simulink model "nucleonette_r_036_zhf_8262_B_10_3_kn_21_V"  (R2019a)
settings: Solver=VariableStepAuto  StartTime=0.0  StopTime=727544.216  FixedStep=0.2  RelTol=1e-6
libraries: simulink x6
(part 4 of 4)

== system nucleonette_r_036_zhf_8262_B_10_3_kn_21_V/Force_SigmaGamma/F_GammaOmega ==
  In1 : Inport
  Add31 : Sum  Inputs=+++
  Add40 : Sum
  Add51 : Sum
  C_10 : Constant  Value=10
  C_100 : Constant  Value=-100
  C_10_11 : Constant  Value=1E-21
  Clock1 : Clock
  Constant : Constant  Value=3
  Constant1 : Constant  Value=2
  Constant15 : Constant  Value=1.0E-3
  Constant24 : Constant  Value=3
  Math Function{1,4,27,30} (4 alike) : Math  Operator=square
  Math Function32 : Math  Operator=pow
  Math Function37 : Math  Operator=pow
  Math Function45 : Math  Operator=pow
  NGamOmex/DGamOmex_3 : Scope
  Omega_w1 : Constant  Value=0.00003453723537
  Product1 : Product  Inputs=*/
  Product{3..4,6..7,12,45,57..58,60} (9 alike) : Product
  Product2 : Product  Inputs=*/
  Product26 : Product  Inputs=*/
  Product31 : Product  Inputs=/**
  Product33 : Product  Inputs=/**
  Product44 : Product  Inputs=**
  Sqrt13 : Sqrt
  Sqrt4 : Sqrt
  Subtract3 : Sum  Inputs=+--
  Subtract4 : Sum
  Trigonometric Function9 : Trigonometry
  ex : Constant  Value=1.602176565
  keGamOmex : Constant  Value=7.39283526
  mSigGamx : Constant  Value=366.300038182
  rx1 : Constant  Value=0.36373
  Out1 : Outport
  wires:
  Math Function1/1 -> Add31/2  "XGO"
  Subtract3/1 -> Product60/2  "Zx_GamOme"
  Product1/1 -> Product3/1, Product7/1  "3/2"
  Omega_w1/1 -> Product57/2
  rx1/1 -> Subtract4/2, Product6/2, Product4/2, Product33/1  "rx"
  Product33/1 -> Math Function37/2
  Math Function32/1 -> Add51/2
  Math Function45/1 -> Add51/1
  Product60/1 -> Product26/1
  C_10/1 -> Math Function37/1
  Constant24/1 -> Math Function45/2, Math Function32/2
  Product57/1 -> Trigonometric Function9/1  "angle_wt"
  Trigonometric Function9/1 -> Product4/1  "sin(wt)"
  Product31/1 -> Product45/2
  Product58/1 -> Math Function27/1  "r*sin(wt)*sqrt(3)/2"
  Product6/1 -> Subtract3/2  "r*sqrt(3)/2"
  Math Function4/1 -> Product31/2
  Product26/1 -> Out1/1, NGamOmex/DGamOmex_3/1  "F_GamOme"
  Clock1/1 -> Product57/1
  Add51/1 -> Product26/2  "DGamOme_B"
  Product45/1 -> Product60/1
  Product4/1 -> Product58/2, Product7/2, Product12/1  "r*sin(wt)"
  Sqrt4/1 -> Product33/2, Math Function32/1  "DGamOme"
  Constant15/1 -> Math Function45/1
  ex/1 -> Math Function4/1
  Constant1/1 -> Product1/2, Product2/2
  Subtract4/1 -> Math Function30/1  "YGamOme"
  Product3/1 -> Subtract3/3  "3z6/2"
  mSigGamx/1 -> Product31/1  "mx"
  Product2/1 -> Product58/1, Product6/1, Product12/2  "sqrt(3)/2"
  Add40/1 -> Product45/1  "kn_DGamOme"
  Constant/1 -> Product1/1, Sqrt13/1
  Math Function37/1 -> Add40/1  "10_exp(-100Dgo/r)"
  C_100/1 -> Product33/3
  Sqrt13/1 -> Product44/2, Product2/1  "sqrt(3)"
  Product12/1 -> Subtract3/1  "r*sin(wt)*sqrt(3)/2"
  C_10_11/1 -> Add40/2
  In1/1 -> Product3/2, Product44/1  "z6"
  Math Function30/1 -> Add31/3
  keGamOmex/1 -> Product31/3
  Math Function27/1 -> Add31/1  "ZGO"
  Add31/1 -> Sqrt4/1
  Product7/1 -> Math Function1/1  "r*sin(wt)3/2"
  Product44/1 -> Subtract4/1  "z6*sqrt(3)"

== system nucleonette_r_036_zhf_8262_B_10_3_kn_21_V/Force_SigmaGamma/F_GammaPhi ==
  In1 : Inport
  Add31 : Sum  Inputs=+++
  Add40 : Sum
  Add51 : Sum
  C_10 : Constant  Value=10
  C_100 : Constant  Value=-100
  C_10_11 : Constant  Value=1E-21
  Clock1 : Clock
  Constant : Constant  Value=3
  Constant1 : Constant  Value=2
  Constant15 : Constant  Value=1.0E-3
  Constant24 : Constant  Value=3
  Math Function{1,4,27,30} (4 alike) : Math  Operator=square
  Math Function32 : Math  Operator=pow
  Math Function37 : Math  Operator=pow
  Math Function45 : Math  Operator=pow
  NGamPhix/DGamPhix_3 : Scope
  Omega_w1 : Constant  Value=0.00003453723537
  Product1 : Product  Inputs=*/
  Product{3..6,12,45,57..58,60} (9 alike) : Product
  Product2 : Product  Inputs=*/
  Product26 : Product  Inputs=*/
  Product31 : Product  Inputs=/**
  Product33 : Product  Inputs=/**
  Product44 : Product  Inputs=**
  Sqrt13 : Sqrt
  Sqrt4 : Sqrt
  Subtract3 : Sum  Inputs=+++
  Subtract4 : Sum  Inputs=+++
  Trigonometric Function10 : Trigonometry  Operator=cos
  Trigonometric Function9 : Trigonometry
  ex : Constant  Value=1.602176565
  keGamPhix : Constant  Value=7.39283526
  mSigGamx : Constant  Value=366.300038182
  rx1 : Constant  Value=0.36373
  Out1 : Outport
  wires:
  Product12/1 -> Subtract3/1  "r*sin(wt)*sqrt(3)/2"
  C_100/1 -> Product33/3
  Constant/1 -> Product1/1, Sqrt13/1
  mSigGamx/1 -> Product31/1  "mx"
  Product3/1 -> Subtract3/3  "3z6/2"
  Subtract4/1 -> Math Function30/1  "YGamPhi"
  Constant1/1 -> Product1/2, Product2/2
  ex/1 -> Math Function4/1
  Constant15/1 -> Math Function45/1
  Sqrt4/1 -> Product33/2, Math Function32/1  "DGamPhi"
  Product4/1 -> Subtract4/1, Product12/1  "r*sin(wt)"
  Product2/1 -> Product6/1, Product12/2  "sqrt(3)/2"
  Product45/1 -> Product60/1
  Add51/1 -> Product26/2  "DGamPhi_B"
  Clock1/1 -> Product57/1
  Product26/1 -> Out1/1, NGamPhix/DGamPhix_3/1  "F_GamPhi"
  Math Function4/1 -> Product31/2
  Product6/1 -> Subtract3/2  "r*sqrt(3)/2"
  Product58/1 -> Math Function27/1  "r*cos(wt)*sqrt(3)"
  Omega_w1/1 -> Product57/2
  Product1/1 -> Product3/1  "3/2"
  Subtract3/1 -> Product60/2  "Zx_GamPhi"
  Math Function1/1 -> Add31/2  "XGP"
  Product33/1 -> Math Function37/2
  Math Function32/1 -> Add51/2
  rx1/1 -> Subtract4/3, Product5/2, Product6/2, Product4/2, Product33/1  "rx"
  Math Function37/1 -> Add40/1  "10_exp(-100Dgp/r)"
  C_10_11/1 -> Add40/2
  Math Function45/1 -> Add51/1
  Add40/1 -> Product45/1  "kn_DGamPhi"
  C_10/1 -> Math Function37/1
  Sqrt13/1 -> Product58/1, Product44/2, Product2/1  "sqrt(3)"
  Product60/1 -> Product26/1
  Math Function27/1 -> Add31/1  "ZGP"
  Trigonometric Function10/1 -> Product5/1  "cos(wt)"
  Math Function30/1 -> Add31/3
  Constant24/1 -> Math Function32/2, Math Function45/2
  In1/1 -> Product3/2, Product44/1  "z6"
  Trigonometric Function9/1 -> Product4/1  "sin(wt)"
  Product31/1 -> Product45/2
  Add31/1 -> Sqrt4/1
  Product57/1 -> Trigonometric Function10/1, Trigonometric Function9/1  "angle_wt"
  keGamPhix/1 -> Product31/3
  Product5/1 -> Product58/2, Math Function1/1  "r*cos(wt)"
  Product44/1 -> Subtract4/2  "z6*sqrt(3)"

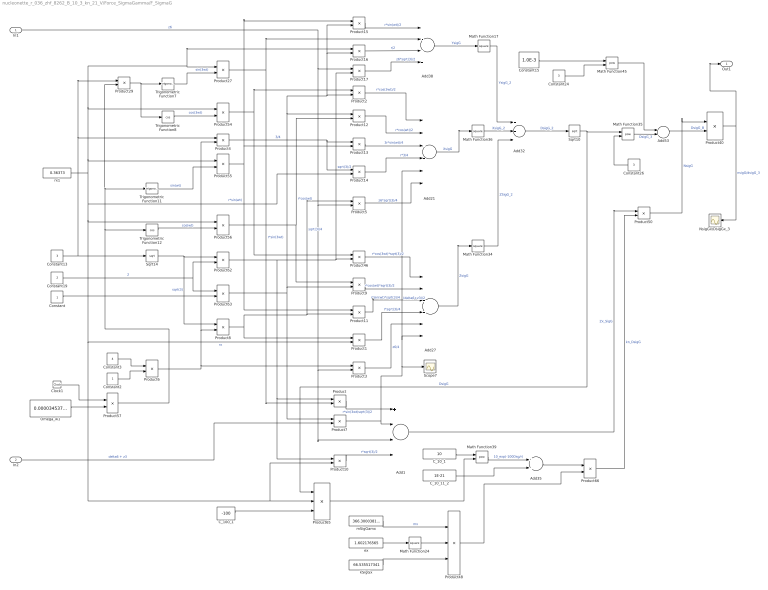
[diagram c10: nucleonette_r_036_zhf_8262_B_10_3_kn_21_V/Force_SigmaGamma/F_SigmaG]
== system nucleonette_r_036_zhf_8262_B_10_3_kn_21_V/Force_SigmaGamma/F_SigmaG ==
  In1 : Inport
  In2 : Inport  Port=2
  Add1 : Sum  Inputs=+---
  Add21 : Sum  Inputs=-+----
  Add27 : Sum  Inputs=-+++++
  Add32 : Sum  Inputs=+++
  Add35 : Sum
  Add38 : Sum  Inputs=--++
  Add53 : Sum
  C_100_1 : Constant  Value=-100
  C_10_1 : Constant  Value=10
  C_10_11_2 : Constant  Value=1E-21
  Clock1 : Clock
  Constant : Constant
  Constant13 : Constant  Value=3
  Constant15 : Constant  Value=1.0E-3
  Constant19 : Constant  Value=2
  Constant2 : Constant
  Constant24 : Constant  Value=3
  Constant26 : Constant  Value=3
  Constant3 : Constant  Value=4
  Math Function{17,24,34,36} (4 alike) : Math  Operator=square
  Math Function35 : Math  Operator=pow
  Math Function39 : Math  Operator=pow
  Math Function45 : Math  Operator=pow
  NsigGx/DsigGx_3 : Scope
  Omega_w1 : Constant  Value=0.00003453723537
  Product{,1..5,7..17,29,46,50,57} (21 alike) : Product
  Product{27,54..56,66} (5 alike) : Product  Inputs=**
  Product40 : Product  Inputs=*/
  Product48 : Product  Inputs=/**
  Product6 : Product  Inputs=/*
  Product62 : Product  Inputs=*/
  Product63 : Product  Inputs=/*
  Product65 : Product  Inputs=*/*
  Scope7 : Scope
  Sqrt10 : Sqrt
  Sqrt14 : Sqrt
  Trigonometric Function11 : Trigonometry
  Trigonometric Function12 : Trigonometry  Operator=cos
  Trigonometric Function7 : Trigonometry
  Trigonometric Function8 : Trigonometry  Operator=cos
  ex : Constant  Value=1.602176565
  kSigGx : Constant  Value=66.535517341
  mSigGamx : Constant  Value=366.300038182
  rx1 : Constant  Value=0.36373
  Out1 : Outport
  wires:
  Add32/1 -> Sqrt10/1  "DsigG_2"
  Add1/1 -> Product50/1  "Zx_SigG"
  Product46/1 -> Add27/1  "r*cos(3wt)*sqrt(3)/2"
  Product62/1 -> Product10/1, Product/1, Product17/2, Product46/2  "sqrt(3)/2"
  Product/1 -> Add1/1  "r*sin(3wt)sqrt(3)/2"
  Product9/1 -> Add27/2  "r*cos(wt)*sqrt(3)/2"
  Math Function45/1 -> Add53/1
  Product29/1 -> Trigonometric Function8/1, Trigonometric Function7/1
  Add53/1 -> Product40/2  "DsigG_B"
  Add27/1 -> Math Function34/1  "ZsigG"
  Product8/1 -> Product11/2, Product5/1, Product1/1  "sqrt(3)/4"
  Constant3/1 -> Product6/1
  Product1/1 -> Add27/4  "r*sqrt(3)/4"
  Add38/1 -> Math Function17/1  "YsigG"
  Product11/1 -> Add27/3  "r*sin(wt)*sqrt(3)/4"
  Product56/1 -> Product12/2, Product9/1  "r*cos(wt)"
  Math Function34/1 -> Add32/3  "ZSigG_2"
  Product55/1 -> Product15/1, Product13/2, Product11/1  "r*sin(wt)"
  Product48/1 -> Product66/2
  Math Function36/1 -> Add32/2  "XsigG_2"
  Constant26/1 -> Math Function35/2
  Product63/1 -> Product12/1, Product2/2, Product15/2, Product16/2, Product9/2, Product7/1
  Product2/1 -> Add21/1  "r*cos(3wt)/2"
  Add35/1 -> Product66/1
  Product13/1 -> Add21/3  "3r*sin(wt)/4"
  Omega_w1/1 -> Product57/2
  Math Function17/1 -> Add32/1  "YsigG_2"
  Product5/1 -> Add21/6  "z6*sqrt(3)/4"
  Product54/1 -> Product2/1, Product46/1
  Product66/1 -> Product50/2  "kn_DsigG"
  Math Function39/1 -> Add35/1  "10_exp(-100Dsg/r)"
  Product12/1 -> Add21/2  "r*cos(wt)/2"
  Product14/1 -> Add21/4  "r*3/4"
  Constant13/1 -> Product4/1, Product29/1, Sqrt14/1
  Trigonometric Function8/1 -> Product54/2  "cos(3wt)"
  In2/1 -> Product7/2  "delta6 + z3"
  Trigonometric Function7/1 -> Product27/2  "sin(3wt)"
  Product7/1 -> Add1/2, Scope7/1, Add21/5, Add27/6  "(delta6+z3)/2"
  Trigonometric Function12/1 -> Product56/2  "cos(wt)"
  Math Function35/1 -> Add53/2  "DsigG_3"
  Product16/1 -> Add38/3  "r/2"
  Product6/1 -> Product4/2, Product8/2, Product3/1
  Product15/1 -> Add38/1  "r*sin(wt)/2"
  Constant19/1 -> Product63/1, Product62/2  "2"
  Product17/1 -> Add38/4  "z6*sqrt(3)/2"
  In1/1 -> Add1/3, Product3/2, Product5/2, Product17/1  "z6"
  Product3/1 -> Add27/5  "z6/4"
  Sqrt10/1 -> Product65/1, Math Function35/1  "DsigG"
  mSigGamx/1 -> Product48/1  "mx"
  Product40/1 -> NsigGx/DsigGx_3/1, Out1/1  "nsigG/dsigG_3"
  Math Function24/1 -> Product48/2
  Trigonometric Function11/1 -> Product55/2  "sin(wt)"
  Product65/1 -> Math Function39/2
  Constant15/1 -> Math Function45/1
  Constant24/1 -> Math Function45/2
  kSigGx/1 -> Product48/3
  Product4/1 -> Product13/1, Product14/1  "3/4"
  rx1/1 -> Product16/1, Product27/1, Product54/1, Product55/1, Product14/2, Product1/2, Product10/2, Product65/2, Product56/1  "rx"
  ex/1 -> Math Function24/1
  Product27/1 -> Add38/2, Product/2  "r*sin(3wt)"
  Product50/1 -> Product40/1  "NsigG"
  C_10_1/1 -> Math Function39/1
  Constant/1 -> Product63/2
  Product57/1 -> Trigonometric Function12/1, Product29/2, Trigonometric Function11/1
  Clock1/1 -> Product57/1
  C_10_11_2/1 -> Add35/2
  C_100_1/1 -> Product65/3
  Add21/1 -> Math Function36/1  "XsigG"
  Sqrt14/1 -> Product62/1, Product8/1  "sqrt(3)"
  Constant2/1 -> Product6/2
  Product10/1 -> Add1/4  "r*sqrt(3)/2"

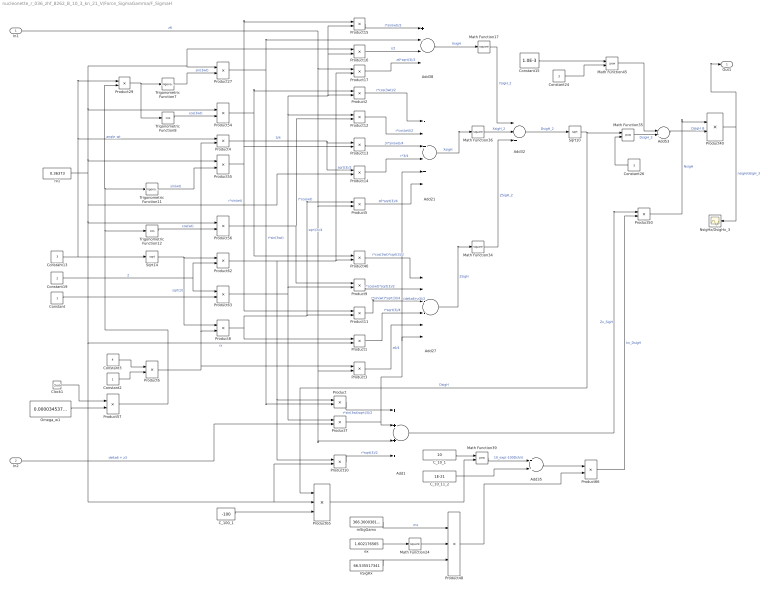
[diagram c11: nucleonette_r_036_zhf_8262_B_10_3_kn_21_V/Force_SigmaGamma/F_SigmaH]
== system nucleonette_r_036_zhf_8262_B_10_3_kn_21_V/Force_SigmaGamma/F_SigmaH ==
  In1 : Inport
  In2 : Inport  Port=2
  Add1 : Sum  Inputs=++++
  Add21 : Sum  Inputs=--++++
  Add27 : Sum  Inputs=------
  Add32 : Sum  Inputs=+++
  Add35 : Sum
  Add38 : Sum  Inputs=+---
  Add53 : Sum
  C_100_1 : Constant  Value=-100
  C_10_1 : Constant  Value=10
  C_10_11_2 : Constant  Value=1E-21
  Clock1 : Clock
  Constant : Constant
  Constant13 : Constant  Value=3
  Constant15 : Constant  Value=1.0E-3
  Constant19 : Constant  Value=2
  Constant2 : Constant
  Constant24 : Constant  Value=3
  Constant26 : Constant  Value=3
  Constant3 : Constant  Value=4
  Math Function{17,24,34,36} (4 alike) : Math  Operator=square
  Math Function35 : Math  Operator=pow
  Math Function39 : Math  Operator=pow
  Math Function45 : Math  Operator=pow
  NsigHx/DsigHx_3 : Scope
  Omega_w1 : Constant  Value=0.00003453723537
  Product{,1..5,7..17,29,46,50,57} (21 alike) : Product
  Product{27,54..56,66} (5 alike) : Product  Inputs=**
  Product40 : Product  Inputs=*/
  Product48 : Product  Inputs=/**
  Product6 : Product  Inputs=/*
  Product62 : Product  Inputs=*/
  Product63 : Product  Inputs=/*
  Product65 : Product  Inputs=*/*
  Sqrt10 : Sqrt
  Sqrt14 : Sqrt
  Trigonometric Function11 : Trigonometry
  Trigonometric Function12 : Trigonometry  Operator=cos
  Trigonometric Function7 : Trigonometry
  Trigonometric Function8 : Trigonometry  Operator=cos
  ex : Constant  Value=1.602176565
  kSigHx : Constant  Value=66.535517341
  mSigGamx : Constant  Value=366.300038182
  rx1 : Constant  Value=0.36373
  Out1 : Outport
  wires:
  Math Function34/1 -> Add32/3  "ZSigH_2"
  Product63/1 -> Product12/1, Product2/2, Product15/2, Product16/2, Product9/2, Product7/1
  Math Function36/1 -> Add32/2  "XsigH_2"
  Product66/1 -> Product50/2  "kn_DsigH"
  Product54/1 -> Product2/1, Product46/1
  Add35/1 -> Product66/1
  Product2/1 -> Add21/1  "r*cos(3wt)/2"
  Math Function17/1 -> Add32/1  "YsigH_2"
  Product55/1 -> Product15/1, Product13/2, Product11/1  "r*sin(wt)"
  Product11/1 -> Add27/3  "r*sin(wt)*sqrt(3)/4"
  Math Function39/1 -> Add35/1  "10_exp(-100Dsh/r)"
  Product5/1 -> Add21/6  "z6*sqrt(3)/4"
  Trigonometric Function7/1 -> Product27/2  "sin(3wt)"
  Trigonometric Function8/1 -> Product54/2  "cos(3wt)"
  Product14/1 -> Add21/4  "r*3/4"
  Constant13/1 -> Product4/1, Product29/1, Sqrt14/1
  In2/1 -> Product7/2  "delta6 + z3"
  Omega_w1/1 -> Product57/2
  Product48/1 -> Product66/2
  Product13/1 -> Add21/3  "3r*sin(wt)/4"
  Product8/1 -> Product11/2, Product5/1, Product1/1  "sqrt(3)/4"
  Add32/1 -> Sqrt10/1  "DsigH_2"
  Product1/1 -> Add27/4  "r*sqrt(3)/4"
  Product62/1 -> Product/1, Product10/1, Product17/2, Product46/2  "sqrt(3)/2"
  Product9/1 -> Add27/2  "r*cos(wt)*sqrt(3)/2"
  Add27/1 -> Math Function34/1  "ZsigH"
  Math Function45/1 -> Add53/1
  Add53/1 -> Product40/2  "DsigH_B"
  Product29/1 -> Trigonometric Function8/1, Trigonometric Function7/1
  Add38/1 -> Math Function17/1  "XsigH"
  Constant3/1 -> Product6/1
  kSigHx/1 -> Product48/3
  Math Function24/1 -> Product48/2
  Sqrt14/1 -> Product62/1, Product8/1  "sqrt(3)"
  Product3/1 -> Add27/5  "z6/4"
  Constant/1 -> Product63/2
  Constant24/1 -> Math Function45/2
  Product57/1 -> Trigonometric Function12/1, Product29/2, Trigonometric Function11/1  "angle_wt"
  Add21/1 -> Math Function36/1  "XsigH"
  Add1/1 -> Product50/1  "Zx_SigH"
  Product17/1 -> Add38/4  "z6*sqrt(3)/2"
  Constant19/1 -> Product63/1, Product62/2  "2"
  Product56/1 -> Product12/2, Product9/1  "r*cos(wt)"
  Product16/1 -> Add38/3  "r/2"
  Trigonometric Function11/1 -> Product55/2  "sin(wt)"
  Clock1/1 -> Product57/1
  Sqrt10/1 -> Product65/1, Math Function35/1  "DsigH"
  mSigGamx/1 -> Product48/1  "mx"
  Product40/1 -> NsigHx/DsigHx_3/1, Out1/1  "nsigH/dsigH_3"
  Trigonometric Function12/1 -> Product56/2  "cos(wt)"
  Product27/1 -> Add38/2, Product/2  "r*sin(3wt)"
  C_100_1/1 -> Product65/3
  Constant26/1 -> Math Function35/2
  Product65/1 -> Math Function39/2
  Constant15/1 -> Math Function45/1
  Product4/1 -> Product13/1, Product14/1  "3/4"
  Constant2/1 -> Product6/2
  Product6/1 -> Product4/2, Product8/2, Product3/1
  Product50/1 -> Product40/1  "NsigH"
  Product12/1 -> Add21/2  "r*cos(wt)/2"
  C_10_1/1 -> Math Function39/1
  ex/1 -> Math Function24/1
  Product/1 -> Add1/1  "r*sin(3wt)sqrt(3)/2"
  Product7/1 -> Add1/2, Add21/5, Add27/6  "(delta6+z3)/2"
  Product46/1 -> Add27/1  "r*cos(3wt)*sqrt(3)/2"
  Math Function35/1 -> Add53/2  "DsigH_3"
  rx1/1 -> Product16/1, Product27/1, Product54/1, Product55/1, Product14/2, Product1/2, Product10/2, Product65/2, Product56/1  "rx"
  In1/1 -> Add1/3, Product3/2, Product5/2, Product17/1  "z6"
  Product15/1 -> Add38/1  "r*sin(wt)/2"
  C_10_11_2/1 -> Add35/2
  Product10/1 -> Add1/4  "r*sqrt(3)/2"

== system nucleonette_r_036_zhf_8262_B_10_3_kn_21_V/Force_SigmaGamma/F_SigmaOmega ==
  In1 : Inport
  Add31 : Sum  Inputs=+++
  Add40 : Sum
  Add51 : Sum
  C_10 : Constant  Value=10
  C_100 : Constant  Value=-100
  C_10_11 : Constant  Value=1E-21
  Clock1 : Clock
  Constant : Constant  Value=3
  Constant1 : Constant  Value=2
  Constant15 : Constant  Value=1.0E-3
  Constant24 : Constant  Value=3
  Math Function{1,4,27,30} (4 alike) : Math  Operator=square
  Math Function32 : Math  Operator=pow
  Math Function37 : Math  Operator=pow
  Math Function45 : Math  Operator=pow
  NSigOmex/DSigOmex_3 : Scope
  Omega_w1 : Constant  Value=0.00003453723537
  Product1 : Product  Inputs=*/
  Product{3..6,12,45,57..58,60} (9 alike) : Product
  Product2 : Product  Inputs=*/
  Product26 : Product  Inputs=*/
  Product31 : Product  Inputs=/**
  Product33 : Product  Inputs=/**
  Product44 : Product  Inputs=**
  Sqrt13 : Sqrt
  Sqrt4 : Sqrt
  Subtract3 : Sum  Inputs=+--
  Subtract4 : Sum  Inputs=-++
  Trigonometric Function10 : Trigonometry  Operator=cos
  Trigonometric Function9 : Trigonometry
  ex : Constant  Value=1.602176565
  keSigOmex : Constant  Value=7.39283526
  mSigGamx : Constant  Value=366.300038182
  rx1 : Constant  Value=0.36373
  Out1 : Outport
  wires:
  Product2/1 -> Product6/1, Product12/2  "sqrt(3)/2"
  Product26/1 -> Out1/1, NSigOmex/DSigOmex_3/1  "F_SigOme"
  Add51/1 -> Product26/2  "DSigOme_B"
  Product6/1 -> Subtract3/2  "r*sqrt(3)/2"
  Subtract4/1 -> Math Function30/1  "YSigOme"
  Constant24/1 -> Math Function45/2, Math Function32/2
  Clock1/1 -> Product57/1
  Constant1/1 -> Product1/2, Product2/2
  Math Function4/1 -> Product31/2
  Product4/1 -> Subtract4/1, Product12/1  "r*sin(wt)"
  In1/1 -> Product3/2, Product44/1  "z6"
  Product31/1 -> Product45/2
  C_10/1 -> Math Function37/1
  Product57/1 -> Trigonometric Function10/1, Trigonometric Function9/1  "angle_wt"
  mSigGamx/1 -> Product31/1  "mx"
  ex/1 -> Math Function4/1
  Trigonometric Function9/1 -> Product4/1  "sin(wt)"
  Product3/1 -> Subtract3/3  "3z6/2"
  Constant15/1 -> Math Function45/1
  Trigonometric Function10/1 -> Product5/1  "cos(wt)"
  Product58/1 -> Math Function27/1  "r*cos(wt)*sqrt(3)"
  Sqrt13/1 -> Product44/2, Product58/1, Product2/1  "sqrt(3)"
  Product12/1 -> Subtract3/1  "r*sin(wt)*sqrt(3)/2"
  Constant/1 -> Product1/1, Sqrt13/1
  C_100/1 -> Product33/3
  Math Function27/1 -> Add31/1  "ZSO"
  keSigOmex/1 -> Product31/3
  Add31/1 -> Sqrt4/1
  C_10_11/1 -> Add40/2
  rx1/1 -> Subtract4/3, Product5/2, Product6/2, Product4/2, Product33/1  "rx"
  Product45/1 -> Product60/1
  Subtract3/1 -> Product60/2  "Zx_SigOme"
  Add40/1 -> Product45/1  "kn_DSigOme"
  Math Function37/1 -> Add40/1  "10_exp(-100Dso/r)"
  Math Function45/1 -> Add51/1
  Sqrt4/1 -> Product33/2, Math Function32/1  "DSigOme"
  Product60/1 -> Product26/1
  Math Function32/1 -> Add51/2
  Product33/1 -> Math Function37/2
  Omega_w1/1 -> Product57/2
  Product1/1 -> Product3/1  "3/2"
  Math Function30/1 -> Add31/3
  Math Function1/1 -> Add31/2  "XSO"
  Product5/1 -> Product58/2, Math Function1/1  "r*cos(wt)"
  Product44/1 -> Subtract4/2  "z6*sqrt(3)"

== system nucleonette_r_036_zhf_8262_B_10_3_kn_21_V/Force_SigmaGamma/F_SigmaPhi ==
  In1 : Inport
  Add31 : Sum  Inputs=+++
  Add40 : Sum
  Add51 : Sum
  C_10 : Constant  Value=10
  C_100 : Constant  Value=-100
  C_10_11 : Constant  Value=1E-21
  Clock1 : Clock
  Constant : Constant  Value=3
  Constant1 : Constant  Value=2
  Constant15 : Constant  Value=1.0E-3
  Constant24 : Constant  Value=3
  Math Function{1,4,27,30} (4 alike) : Math  Operator=square
  Math Function32 : Math  Operator=pow
  Math Function37 : Math  Operator=pow
  Math Function45 : Math  Operator=pow
  NSigPhix/DSigPhix_3 : Scope
  Omega_w1 : Constant  Value=0.00003453723537
  Product1 : Product  Inputs=*/
  Product{3..4,6..7,12,45,57..58,60} (9 alike) : Product
  Product2 : Product  Inputs=*/
  Product26 : Product  Inputs=*/
  Product31 : Product  Inputs=/**
  Product33 : Product  Inputs=/**
  Product44 : Product  Inputs=**
  Sqrt13 : Sqrt
  Sqrt4 : Sqrt
  Subtract3 : Sum  Inputs=+++
  Subtract4 : Sum
  Trigonometric Function9 : Trigonometry
  ex : Constant  Value=1.602176565
  keSigPhix : Constant  Value=7.39283526
  mSigGamx : Constant  Value=366.300038182
  rx1 : Constant  Value=0.36373
  Out1 : Outport
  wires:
  Math Function1/1 -> Add31/2  "XSP"
  Subtract3/1 -> Product60/2  "Zx_SigPhi"
  Product1/1 -> Product3/1, Product7/2  "3/2"
  Omega_w1/1 -> Product57/2
  rx1/1 -> Product33/1, Subtract4/2, Product6/2, Product4/2  "rx"
  Product33/1 -> Math Function37/2
  Math Function32/1 -> Add51/2
  Math Function45/1 -> Add51/1
  Product60/1 -> Product26/1
  C_10/1 -> Math Function37/1
  Constant24/1 -> Math Function32/2, Math Function45/2
  Product57/1 -> Trigonometric Function9/1  "angle_wt"
  Trigonometric Function9/1 -> Product4/1  "sin(wt)"
  Product31/1 -> Product45/2
  Product58/1 -> Math Function27/1  "r*sin(wt)*sqrt(3)/2"
  Product6/1 -> Subtract3/2  "r*sqrt(3)/2"
  Math Function4/1 -> Product31/2
  Product26/1 -> Out1/1, NSigPhix/DSigPhix_3/1  "F_SigPhi"
  Clock1/1 -> Product57/1
  Product44/1 -> Subtract4/1  "z6*sqrt(3)"
  Add51/1 -> Product26/2  "DSigPhi_B"
  Product45/1 -> Product60/1
  Product2/1 -> Product58/2, Product6/1, Product12/2  "sqrt(3)/2"
  Product4/1 -> Product7/1, Product58/1, Product12/1  "r*sin(wt)"
  Sqrt4/1 -> Product33/2, Math Function32/1  "DSigPhi"
  Constant15/1 -> Math Function45/1
  ex/1 -> Math Function4/1
  Constant1/1 -> Product1/2, Product2/2
  Subtract4/1 -> Math Function30/1  "YSigPhi"
  Product3/1 -> Subtract3/3  "3z6/2"
  mSigGamx/1 -> Product31/1  "mx"
  Product7/1 -> Math Function1/1  "r*sin(wt)*3/2"
  Constant/1 -> Product1/1, Sqrt13/1
  Math Function37/1 -> Add40/1  "10_exp(-100Dsp/r)"
  C_100/1 -> Product33/3
  Product12/1 -> Subtract3/1  "r*sin(wt)*sqrt(3)/2"
  Sqrt13/1 -> Product44/2, Product2/1  "sqrt(3)"
  C_10_11/1 -> Add40/2
  Add40/1 -> Product45/1  "kn_DSigPhi"
  In1/1 -> Product3/2, Product44/1  "z6"
  Math Function30/1 -> Add31/3
  keSigPhix/1 -> Product31/3
  Math Function27/1 -> Add31/1  "ZSP"
  Add31/1 -> Sqrt4/1
